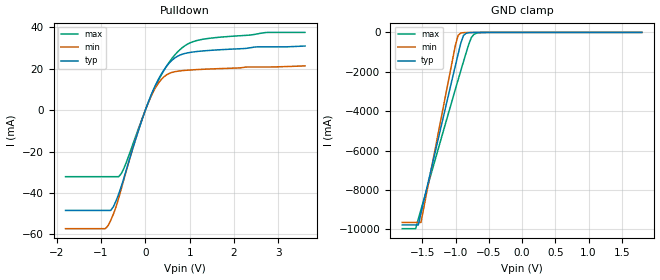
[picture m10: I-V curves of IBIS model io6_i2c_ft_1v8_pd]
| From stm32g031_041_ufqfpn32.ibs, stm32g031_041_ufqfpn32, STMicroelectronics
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|   Model io6_i2c_ft_1v8_pd
[Model]  io6_i2c_ft_1v8_pd
Model_type I/O_open_drain
Polarity   Non-Inverting
Enable   Active-High
Vinl =   0.540000V
Vinh =   1.260000V
Vmeas =  0.900000V
Cref =   30.000000pF
Rref =   100.000000
Vref =   2.000000V
C_comp   1.962900pF   1.853500pF   2.066400pF
[Temperature Range]   25.000000   -40.000000   0.125000k
[Pullup Reference]   1.800000V   1.600000V   2.000000V
[Pulldown Reference]   0.0V   0.0V   0.0V
[POWER Clamp Reference]   1.800000V   1.600000V   2.000000V
[GND Clamp Reference]   0.0V   0.0V   0.0V
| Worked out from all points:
|   slope of the pulldown table from 0 to 0.27 V, typ, clamps not added: 19.5 ohm
|   GND clamp passes 1 mA (typ) near -0.58 V on its own axis
[Pulldown]
|Voltage   I(typ)   I(min)   I(max)
-1.8V     -48.4mA    -57.21mA   -32.11mA
-900mV    -48.4mA    -57.21mA   -32.11mA
-720mV    -46.59mA   -50.17mA   -32.11mA
-600mV    -40.49mA   -42.46mA   -32.11mA
-480mV    -32.55mA   -33.19mA   -27.92mA
0V        5.59pA     4.76pA     350.4pA
240mV     12.61mA    11.25mA    12.03mA
480mV     21.24mA    17.09mA    21.34mA
840mV     27.09mA    19.12mA    30.31mA
1.2V      28.42mA    19.65mA    33.84mA
2.76V     30.59mA    20.86mA    37.58mA
3.6V      30.99mA    21.4mA     37.58mA
[GND_clamp]
|Voltage   I(typ)   I(min)   I(max)
-1.8V     -9.78A     -9.654A    -9.97A
-1.6V     -9.78A     -9.654A    -9.97A
-1.56V    -9.78A     -9.654A    -9.488A
-1.52V    -9.197A    -9.654A    -9.009A
-1V       -1.657A    -623.4mA   -2.861A
-960mV    -1.089A    -143.5mA   -2.397A
-920mV    -532.3mA   -32.25mA   -1.936A
-880mV    -156.3mA   -12.42mA   -1.48A
-840mV    -44.7mA    -7.779mA   -1.031A
-760mV    -8.016mA   -3.95mA    -244.2mA
-680mV    -3.283mA   -1.507mA   -34.99mA
1.8V      0A         0A         0A
[POWER_clamp]
|Voltage   I(typ)   I(min)   I(max)
-1.8V     0A         0A         0A
0V        0A         0A         0A
[Ramp]
| variable   typ   min   max
dV/dt_r  0.72041/0.64222n   0.55729/1.09866n   0.79948/0.66419n
dV/dt_f  0.72041/5.32491n   0.55791/7.70210n   0.79948/4.48839n
R_load = 50.000000
|End [Model] io6_i2c_ft_1v8_pd
